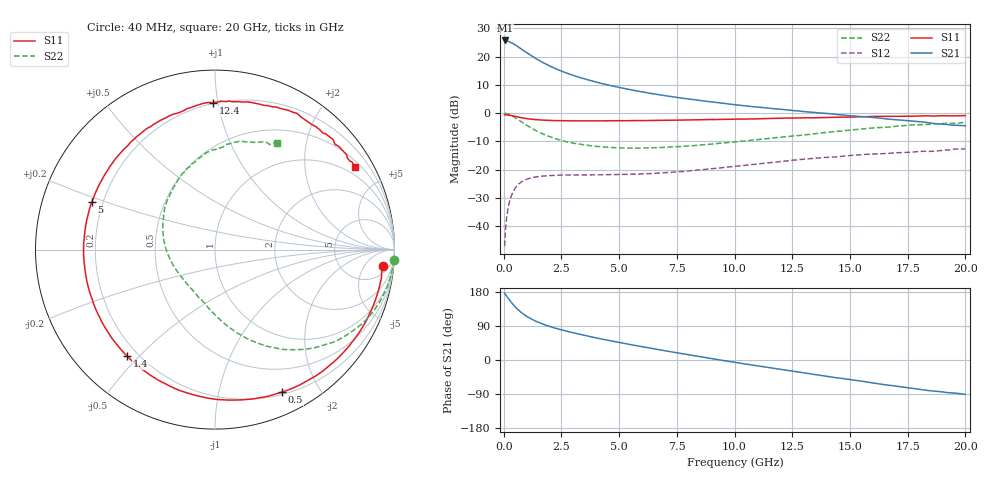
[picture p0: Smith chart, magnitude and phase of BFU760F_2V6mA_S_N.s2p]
! Filename:  P:\Prog\Test\Noise\ATS_data\Testdata_Net\BFU760\BFU760F_2W_C1_2V6mA_D.s2p
! Date/Time: Mon 06/Feb/2012 15:05:10
! BFU760_2W_C1_2V_6mA
! bias mode 1: Vout= 2.0003 V, Iout= 5.9600 mA, Vin= 0.7614 V, Iin= 0.0169 mA
! Date/time Fri Mar 18 12:28:23 2011
! Device data file deembeded for feedlines and parallel
! Original file: \BFU760\BFU760_2W_C1_2V6mA_R.s2p
! Feed-files: PR003V01_101208_Feed1.s2p, PR003V01_101208_Feed2.s2p
! Parallel-file: PR003V01_101208_Par.s2p
# MHz S MA R 50
!  Freq-MHz  S11-mag  S11-arg  S21-mag  S21-arg  S12-mag  S12-arg  S22-mag  S22-arg
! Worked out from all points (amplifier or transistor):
!   167 points, 40 MHz to 20 GHz, reference 50 ohm
!   highest |S21| = 25.7 dB at 50 MHz (marker M1)
!   |S21| within 3 dB of that: start of sweep to 761.9 MHz
!   unconditionally stable (mu >= 1): 5.832 GHz to 12.76 GHz; 12.92 GHz to 13.04 GHz
!   at 550 MHz: K = 0.08, MSG = 24.9 dB, |S12| = -26.0 dB
!   at 4.2 GHz: K = 0.74, MSG = 16.2 dB, |S12| = -21.8 dB
!   at 20 GHz: K = 0.79, MSG = 4.1 dB, |S12| = -12.7 dB
!   lowest NFmin = 0.38 dB at 400 MHz
!   S11 on the Smith chart (normalised r, x): 40 MHz: 9, -15; 500 MHz: 0.23, -1.55; 1.4 GHz: 0.16, -0.46; 5 GHz: 0.16, +0.18; 12.4 GHz: 0.19, +0.97; 20 GHz: 0.68, +3.55
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40  0.9416 -5.7  19.33 176.6  0.004453 85.5  0.9962 -3.4
50  0.9375 -7.6  19.35 175.1  0.005454 89.2  0.9947 -4.2
60  0.9375 -8.1  19.09 174.4  0.006813 86.1  0.9952 -5.0
140  0.9355 -19.5  18.98 167.6  0.01549 79.6  0.9827 -11.8
280  0.9169 -38.3  18.07 155.9  0.02977 69.7  0.9383 -23.0
420  0.8917 -55.8  16.95 145.5  0.04173 60.6  0.874 -33.0
500  0.8775 -64.8  16.12 140.2  0.04736 55.9  0.8338 -38.4
650  0.8503 -80.0  14.7 131.2  0.05587 48.4  0.7584 -46.9
900  0.8137 -100.8  12.48 119.2  0.06541 38.8  0.647 -58.0
1150  0.7875 -116.8  10.68 109.8  0.07119 31.9  0.5591 -66.8
1400  0.7694 -129.4  9.221 102.2  0.07475 26.6  0.4908 -74.0
1750  0.7525 -142.9  7.682 93.6  0.07773 21.4  0.421 -82.0
2150  0.7412 -154.8  6.392 85.5  0.07938 17.2  0.3646 -89.8
2700  0.7347 -167.3  5.175 76.5  0.08065 13.3  0.3135 -98.9
3400  0.7321 -179.6  4.165 66.4  0.08121 10.2  0.2795 -109.4
5000  0.7359 158.7  2.858 46.3  0.08252 7.8  0.2432 -132.7
6800  0.7478 139.7  2.103 26.4  0.0876 8.6  0.2475 -157.8
10200  0.7874 109.0  1.389 -8.0  0.1169 6.3  0.3171 156.6
12400  0.8193 90.7  1.133 -28.4  0.1456 -1.2  0.3898 131.0
13400  0.8296 82.9  1.036 -37.4  0.159 -7.0  0.43 120.1
16800  0.8804 55.8  0.7767 -67.3  0.1966 -27.4  0.5736 85.5
20000  0.9072 30.5  0.6016 -91.0  0.2329 -49.9  0.6859 59.8
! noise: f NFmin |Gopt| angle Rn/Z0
400  0.3821  0.3733  23.63  0.0806
650  0.3907  0.349  39.65  0.0798
1050  0.4081  0.3452  63.57  0.0772
1450  0.4301  0.3641  83.32  0.0731
1850  0.4566  0.3892  99.47  0.0679
2250  0.4876  0.4139  113.4  0.062
3000  0.558  0.4577  136.5  0.0504
3800  0.6507  0.5101  158.4  0.0395
4600  0.7615  0.5705  176.8  0.033
6000  0.9989  0.6353  200.2  0.0411
